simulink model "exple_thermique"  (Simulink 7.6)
settings: Solver=ode15s  StartTime=0.0  StopTime=36000  RelTol=1e-3
InitFcn:
  | T1=55+273.15;             % température à x=0, [K]
  | T0=25+273.15;             % température à x=L (température de l'air ambiant) [K]
  | L=10;                           % épaisseur
  | Lambda=46;                 % conductivité thermique [W/(m*K)]
  | A= 0.7854;                   % surface d'échange [m^2]
  | V=A*L;                        % volume, [m3]
  | M=50;                          % Masse du système, [kg]
  | rho=M/ V;                     % masse volumique, [kg/m^3]
  | C=447;                         % Capacité calorifique, [J/kg/K]
  | a=Lambda/(rho*C);      % diffusivité thermique, [m^2/s]
  | h=10;                          % coefficient d'échange par convection, [W/m^2.K]
  | R1=L/(Lambda*A);       % Résistance conductive
  | R2=1/(h*A);                % Résistance convective
  | Cth=M*C;                    % Capacité thermique du mur
StopFcn:
  | load result.mat
  | plot(x(1,:),x(2,:),x(1,:),x(3,:))
  | title('Température dans le mur et tension aux bornes de la capacité Cth')
  | grid
  | xlabel('temps')
  | 
  | delete *.mat
libraries: fl_lib x16, nesl_utility x6

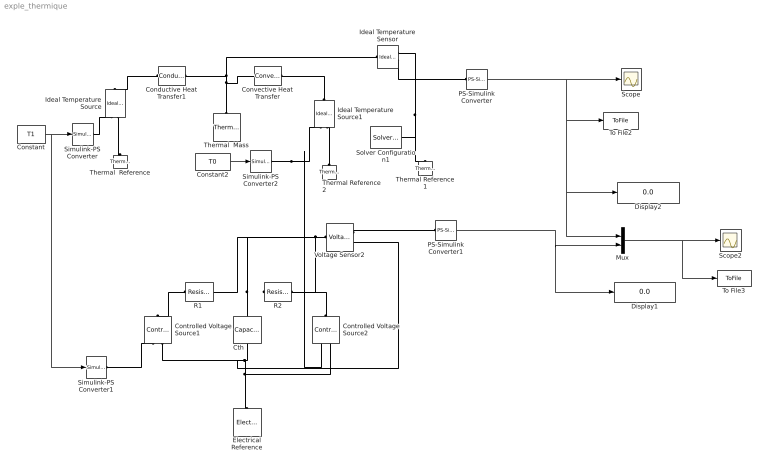
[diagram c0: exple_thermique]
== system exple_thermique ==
  Conductive Heat Transfer1 : fl_lib/Thermal/Thermal Elements/Conductive Heat Transfer  DialogController=NetworkEngine.DynNeDlgSource  SystemSampleTime=-1  area=0.7854 m^2  thickness=x0 m  th_cond=Lambda W/(m*K)  Q_Log=off  T_Log=off  LocalVarNames=|Q|T  LocalVarDescs=|Q|T  LocalVarLogging=[0 0]
  Constant : Constant  Value=T1
  Constant2 : Constant  Value=T0
  Controlled Voltage Source1 : fl_lib/Electrical/Electrical Sources/Controlled Voltage Source  DialogController=NetworkEngine.DynNeDlgSource  SystemSampleTime=-1  i_Log=off  v_Log=off  LocalVarNames=|i|v  LocalVarDescs=|i|v  LocalVarLogging=[0 0]
  Controlled Voltage Source2 : fl_lib/Electrical/Electrical Sources/Controlled Voltage Source  DialogController=NetworkEngine.DynNeDlgSource  SystemSampleTime=-1  i_Log=off  v_Log=off  LocalVarNames=|i|v  LocalVarDescs=|i|v  LocalVarLogging=[0 0]
  Convective Heat Transfer : fl_lib/Thermal/Thermal Elements/Convective Heat Transfer  DialogController=NetworkEngine.DynNeDlgSource  SystemSampleTime=-1  area=A m^2  heat_tr_coeff=h W/(m^2 * K)  Q_Log=off  T_Log=off  LocalVarNames=|Q|T  LocalVarDescs=|Q|T  LocalVarLogging=[0 0]
  Cth : fl_lib/Electrical/Electrical Elements/Capacitor  DialogController=NetworkEngine.DynNeDlgSource  SystemSampleTime=-1  c=Cth F  v0=-T0 V  r=1e-9 Ohm  g=0 1/Ohm  i_Log=off  v_Log=off  vc_Log=off  LocalVarNames=|i|v|vc  LocalVarDescs=|i|v|Internal variable for voltage across capacitor term  LocalVarLogging=[0 0 0]
  Display1 : Display
  Display2 : Display
  Electrical Reference : fl_lib/Electrical/Electrical Elements/Electrical Reference  DialogController=NetworkEngine.DynNeDlgSource  SystemSampleTime=-1  i_Log=off  LocalVarNames=|i  LocalVarDescs=|i  LocalVarLogging=0
  Ideal Temperature Sensor : fl_lib/Thermal/Thermal Sensors/Ideal Temperature Sensor  DialogController=NetworkEngine.DynNeDlgSource  SystemSampleTime=-1  Qs_Log=off  Ts_Log=off  LocalVarNames=|Qs|Ts  LocalVarDescs=|Qs|Ts  LocalVarLogging=[0 0]
  Ideal Temperature Source : fl_lib/Thermal/Thermal Sources/Ideal Temperature Source  DialogController=NetworkEngine.DynNeDlgSource  SystemSampleTime=-1  Q_Log=off  T_Log=off  LocalVarNames=|Q|T  LocalVarDescs=|Q|T  LocalVarLogging=[0 0]
  Ideal Temperature Source1 : fl_lib/Thermal/Thermal Sources/Ideal Temperature Source  DialogController=NetworkEngine.DynNeDlgSource  SystemSampleTime=-1  Q_Log=off  T_Log=off  LocalVarNames=|Q|T  LocalVarDescs=|Q|T  LocalVarLogging=[0 0]
  Mux : Mux  Inputs=2
  PS-Simulink Converter : nesl_utility/PS-Simulink Converter  DialogController=NetworkEngine.DynNeUtilDlgSource  SystemSampleTime=-1  PhysicalDomain=network_engine_domain  LeftPortType=input  RightPortType=output  SubClassName=ps_output  Unit=1  AffineConversion=off
  PS-Simulink Converter1 : nesl_utility/PS-Simulink Converter  DialogController=NetworkEngine.DynNeUtilDlgSource  SystemSampleTime=-1  PhysicalDomain=network_engine_domain  LeftPortType=input  RightPortType=output  SubClassName=ps_output  Unit=1  AffineConversion=off
  "R1 " : fl_lib/Electrical/Electrical Elements/Resistor  DialogController=NetworkEngine.DynNeDlgSource  SystemSampleTime=-1  R=R1 Ohm  i_Log=off  v_Log=off  LocalVarNames=|i|v  LocalVarDescs=|i|v  LocalVarLogging=[0 0]
  R2 : fl_lib/Electrical/Electrical Elements/Resistor  DialogController=NetworkEngine.DynNeDlgSource  SystemSampleTime=-1  R=R2 Ohm  i_Log=off  v_Log=off  LocalVarNames=|i|v  LocalVarDescs=|i|v  LocalVarLogging=[0 0]
  Scope : Scope
  Scope2 : Scope
  Simulink-PS Converter : nesl_utility/Simulink-PS Converter  DialogController=NetworkEngine.DynNeUtilDlgSource  SystemSampleTime=-1  PhysicalDomain=network_engine_domain  LeftPortType=input  RightPortType=output  SubClassName=ps_input  Unit=1  AffineConversion=off  InputFilterTimeConstant=.001  UdotUserProvided=0
  Simulink-PS Converter1 : nesl_utility/Simulink-PS Converter  DialogController=NetworkEngine.DynNeUtilDlgSource  SystemSampleTime=-1  PhysicalDomain=network_engine_domain  LeftPortType=input  RightPortType=output  SubClassName=ps_input  Unit=1  AffineConversion=off  InputFilterTimeConstant=.001  UdotUserProvided=0
  Simulink-PS Converter2 : nesl_utility/Simulink-PS Converter  DialogController=NetworkEngine.DynNeUtilDlgSource  SystemSampleTime=-1  PhysicalDomain=network_engine_domain  LeftPortType=input  RightPortType=output  SubClassName=ps_input  Unit=1  AffineConversion=off  InputFilterTimeConstant=.001  UdotUserProvided=0
  Solver Configuration1 : nesl_utility/Solver Configuration  DialogController=NetworkEngine.DynNeUtilDlgSource  SystemSampleTime=-1  PhysicalDomain=network_engine_domain  LeftPortType=input  RightPortType=generic  SubClassName=solver  Accelerate=off  Profile=off  ResidualTolerance=1e-9  MaxNonlinIter=3  MaxModeIter=2  DoFixedCost=off  UseLocalSampling=off  DoDC=off  LinearAlgebra=Sparse  LocalSolverSampleTime=.001  LocalSolverChoice=NE_BACKWARD_EULER_ADVANCER  UseLocalSolver=off
  Thermal  Mass : fl_lib/Thermal/Thermal Elements/Thermal Mass  DialogController=NetworkEngine.DynNeDlgSource  SystemSampleTime=-1  mass=M kg  sp_heat=C J/kg/K  init_temp=T0 K  Q_Log=off  LocalVarNames=|Q  LocalVarDescs=|Q  LocalVarLogging=0
  Thermal  Reference : fl_lib/Thermal/Thermal Elements/Thermal Reference  DialogController=NetworkEngine.DynNeDlgSource  SystemSampleTime=-1  Q_Log=off  LocalVarNames=|Q  LocalVarDescs=|Q  LocalVarLogging=0
  Thermal Reference1 : fl_lib/Thermal/Thermal Elements/Thermal Reference  DialogController=NetworkEngine.DynNeDlgSource  SystemSampleTime=-1  Q_Log=off  LocalVarNames=|Q  LocalVarDescs=|Q  LocalVarLogging=0
  Thermal Reference2 : fl_lib/Thermal/Thermal Elements/Thermal Reference  DialogController=NetworkEngine.DynNeDlgSource  SystemSampleTime=-1  Q_Log=off  LocalVarNames=|Q  LocalVarDescs=|Q  LocalVarLogging=0
  To File2 : ToFile  Filename=T  MatrixName=z
  To File3 : ToFile  Filename=result  MatrixName=x
  Voltage Sensor2 : fl_lib/Electrical/Electrical Sensors/Voltage Sensor  DialogController=NetworkEngine.DynNeDlgSource  SystemSampleTime=-1  i1_Log=off  v1_Log=off  LocalVarNames=|i1|v1  LocalVarDescs=|i1|v1  LocalVarLogging=[0 0]
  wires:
  Constant/1 -> Simulink-PS Converter/1, Simulink-PS Converter1/1
  PS-Simulink Converter/1 -> Scope/1, To File2/1, Mux/1, Display2/1
  Mux/1 -> Scope2/1, To File3/1
  PS-Simulink Converter1/1 -> Display1/1, Mux/2
  Constant2/1 -> Simulink-PS Converter2/1
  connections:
  Simulink-PS Converter/RConn1 -- Ideal Temperature Source/RConn1
  Ideal Temperature Source/RConn2 -- Thermal  Reference/LConn1
  Convective Heat Transfer/LConn1 -- Conductive Heat Transfer1/RConn1 -- Thermal  Mass/LConn1 -- Ideal Temperature Sensor/LConn1
  Ideal Temperature Sensor/RConn2 -- PS-Simulink Converter/LConn1
  Ideal Temperature Sensor/RConn1 -- Thermal Reference1/LConn1 -- Solver Configuration1/RConn1
  Conductive Heat Transfer1/LConn1 -- Ideal Temperature Source/LConn1
  Voltage Sensor2/LConn1 -- Cth/RConn1 -- "R1 "/RConn1 -- R2/LConn1
  Controlled Voltage Source1/RConn2 -- Cth/LConn1 -- Voltage Sensor2/RConn2 -- Electrical Reference/LConn1 -- Controlled Voltage Source2/RConn2
  Voltage Sensor2/RConn1 -- PS-Simulink Converter1/LConn1
  Simulink-PS Converter1/RConn1 -- Controlled Voltage Source1/RConn1
  "R1 "/LConn1 -- Controlled Voltage Source1/LConn1
  Simulink-PS Converter2/RConn1 -- Ideal Temperature Source1/RConn1 -- Controlled Voltage Source2/RConn1
  Ideal Temperature Source1/LConn1 -- Convective Heat Transfer/RConn1
  Thermal Reference2/LConn1 -- Ideal Temperature Source1/RConn2
  Controlled Voltage Source2/LConn1 -- R2/RConn1
